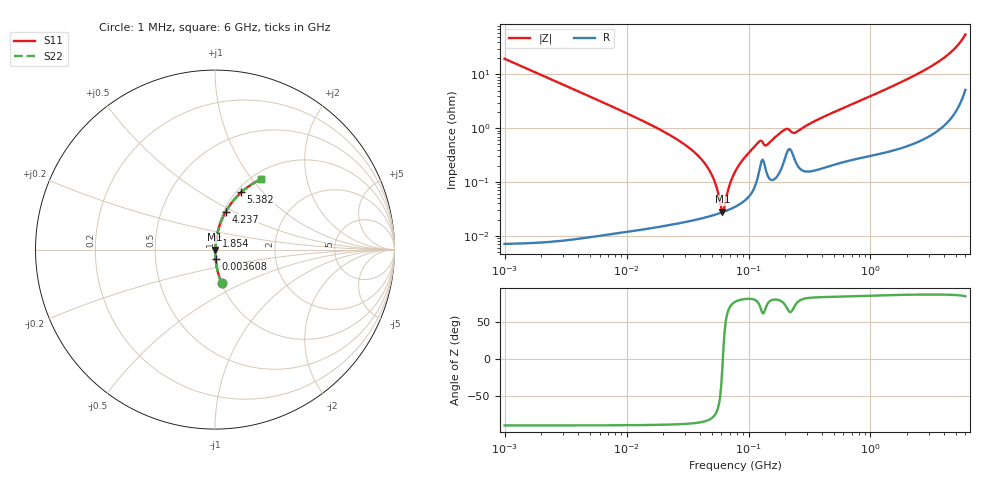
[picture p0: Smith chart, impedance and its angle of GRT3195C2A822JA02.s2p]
!Murata Part Number: GRT3195C2A822JA02
!These Parameters are Measured in Series Mode Connection
!Data Generated on Jun 19, 2026
!  o--ll--o
!Port1  Port2
!  o------o
!Operation Temp=25[degC], DC Bias Voltage=0[V]
!Freq. Start=1000[kHz] Stop=6[GHz] 401[Steps]
# Hz S RI R 50
!Freq.(Hz) S11(Real) S11(Imag) S21(Real) S21(Imag) S12(Real) S12(Imag) S22(Real) S22(Imag)
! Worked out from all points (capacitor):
!   401 points, 1 MHz to 6 GHz, reference 50 ohm
!   read as one part in series: C = 8.12 nF near 1.044 MHz
!   lowest |Z| = 28 mohm at 60.98 MHz (marker M1)
!   series resonance near 61.57 MHz, so ESL is about 820 pH
!   S11 on the Smith chart (normalised r, x): 1 MHz: 1.00, -0.39; 3.608 MHz: 1.00, -0.11; 1.854 GHz: 1.01, +0.15; 4.237 GHz: 1.03, +0.45; 5.382 GHz: 1.06, +0.77; 6 GHz: 1.10, +1.11
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1000000  0.037 -0.1887  0.963 0.1887  0.963 0.1887  0.037 -0.1887
3608090  0.003 -0.054  0.997 0.054  0.997 0.054  0.003 -0.054
4293785  0.00215 -0.0453  0.9979 0.0453  0.9979 0.0453  0.00215 -0.0453
1.843659e7  0.000239 -0.00965  0.9998 0.00965  0.9998 0.00965  0.000239 -0.00965
3.040356e7  0.000204 -0.00486  0.9998 0.00486  0.9998 0.00486  0.000204 -0.00486
4.213132e7  0.000219 -0.00247  0.9998 0.00247  0.9998 0.00247  0.000219 -0.00247
5.124051e7  0.000242 -0.00118  0.9998 0.00118  0.9998 0.00118  0.000242 -0.00118
6.097846e7  0.000273 -6.13e-05  0.9997 6.13e-05  0.9997 6.13e-05  0.000273 -6.13e-05
6.368941e7  0.000284 0.000218  0.9997 -0.000218  0.9997 -0.000218  0.000284 0.000218
6.947823e7  0.000308 0.000782  0.9997 -0.000782  0.9997 -0.000782  0.000308 0.000782
7.745967e7  0.000347 0.00151  0.9997 -0.00151  0.9997 -0.00151  0.000347 0.00151
9.218041e7  0.00045 0.00275  0.9996 -0.00275  0.9996 -0.00275  0.00045 0.00275
1.223006e8  0.00163 0.00542  0.9984 -0.00542  0.9984 -0.00542  0.00163 0.00542
1.424119e8  0.0014 0.00475  0.9986 -0.00475  0.9986 -0.00475  0.0014 0.00475
1.973453e8  0.00266 0.00898  0.9973 -0.00898  0.9973 -0.00898  0.00266 0.00898
2.400133e8  0.00261 0.00781  0.9974 -0.00781  0.9974 -0.00781  0.00261 0.00781
3.325952e8  0.00176 0.0127  0.9982 -0.0127  0.9982 -0.0127  0.00176 0.0127
1.428092e9  0.00686 0.0563  0.9931 -0.0563  0.9931 -0.0563  0.00686 0.0563
1.853962e9  0.0099 0.0741  0.9901 -0.0741  0.9901 -0.0741  0.0099 0.0741
4.236675e9  0.059 0.2094  0.941 -0.2094  0.941 -0.2094  0.059 0.2094
5.38176e9  0.1462 0.3193  0.8538 -0.3193  0.8538 -0.3193  0.1462 0.3193
6e9  0.2549 0.3915  0.7451 -0.3915  0.7451 -0.3915  0.2549 0.3915
